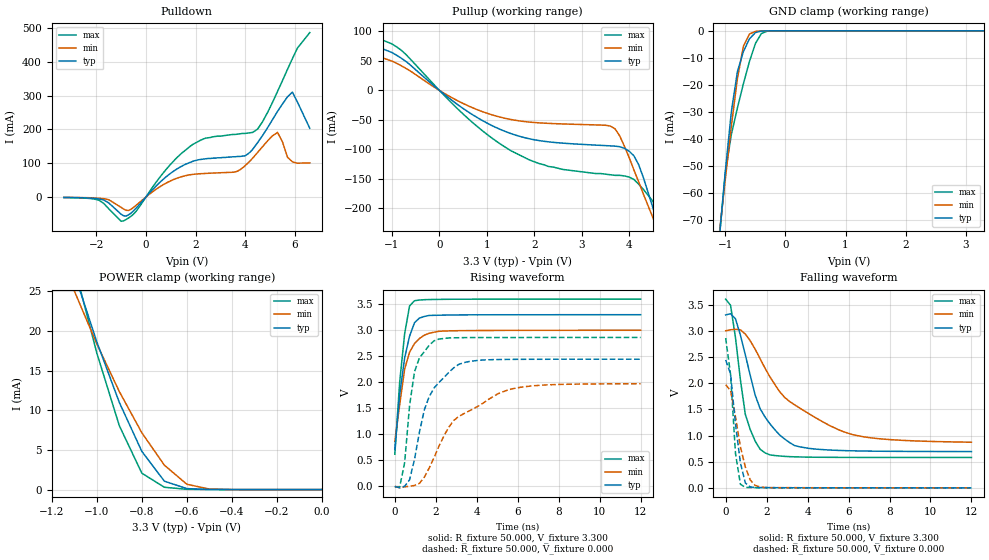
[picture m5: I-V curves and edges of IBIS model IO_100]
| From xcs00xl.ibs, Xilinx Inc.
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|   Model IO_100
[Model]   IO_100
Model_type   I/O
Polarity   Non-Inverting
Enable   Active-Low
Vinl =   0.800V
Vinh =   2.000V
Vmeas =   1.650V
Cref =  50.000pF
Rref =   1.000M
Vref =  0.000V
C_comp   5.300pF   3.500pF   6.800pF
[Temperature Range]   50.000   100.000   0.000
[Voltage Range]   3.300V   3.000V   3.600V
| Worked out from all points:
|   slope of the pulldown table from 0 to 0.495 V, typ, clamps not added: 12.8 ohm
|   slope of the pullup table from 0 to 0.495 V, typ, clamps not added: 16.3 ohm
|   GND clamp passes 1 mA (typ) near -0.52 V on its own axis
|   POWER clamp passes 1 mA (typ) near -0.69 V on its own axis
|   rising waveform, R_fixture 50.000, V_fixture 3.300: 20-80 % time 543ps typ, 571ps min, 408ps max; typ from 0.7 V to 3.3 V
|   rising waveform, R_fixture 50.000, V_fixture 0.000: 20-80 % time 1.12ns typ, 2.49ns min, 534ps max; typ from -0.012 V to 2.44 V
|   falling waveform, R_fixture 50.000, V_fixture 3.300: 20-80 % time 1.37ns typ, 3.04ns min, 712ps max; typ from 3.31 V to 0.694 V
|   falling waveform, R_fixture 50.000, V_fixture 0.000: 20-80 % time 421ps typ, 588ps min, 318ps max; typ from 2.44 V to 0.001 V
[Pulldown]
| voltage   I(typ)   I(min)   I(max)
-3.3V     -1.3mA     -1mA       -1.5mA
-1.9V     -5.4mA     -3.4mA     -9mA
-1V       -50.64mA   -30.43mA   -71.65mA
-700mV    -52.55mA   -39.74mA   -61.89mA
800mV     58.88mA    40.69mA    80.44mA
1.8V      103mA      66.09mA    151mA
3.6V      119mA      74.19mA    185mA
4V        122mA      93.03mA    188mA
4.5V      161mA      132mA      201mA
5.3V      253mA      191mA      312mA
5.9V      310mA      104mA      409mA
6.6V      203mA      101mA      486mA
[Pullup]
| voltage   I(typ)   I(min)   I(max)
-3.3V     5.1mA      940uA      37.2mA
-3.1V     7.54mA     1.17mA     90.7mA
-2.9V     27.6mA     1.66mA     104mA
-2.7V     86.4mA     3.45mA     105mA
-2.3V     90.2mA     70mA       105mA
-1.5V     80.17mA    63.43mA    95.35mA
-800mV    54.4mA     41.67mA    67.93mA
1.5V      -72.97mA   -49.19mA   -102mA
3.7V      -94.47mA   -64.95mA   -144mA
4.1V      -111mA     -135mA     -151mA
4.7V      -250mA     -255mA     -227mA
6.6V      -645mA     -572mA     -737mA
[GND_clamp]
| voltage   I(typ)   I(min)   I(max)
-3.3V     -539mA     -461mA     -635mA
-1.1V     -76.29mA   -74.81mA   -76.3mA
-1V       -51.66mA   -54.6mA    -52.25mA
-900mV    -29.77mA   -35.09mA   -38.23mA
-800mV    -15.1mA    -17.65mA   -28.49mA
-700mV    -7.645mA   -5.66mA    -19.53mA
-600mV    -2.968mA   -1.205mA   -11.34mA
-500mV    -649uA     -202uA     -4.68mA
-400mV    -83.34uA   -28.89uA   -976uA
-300mV    -8.303uA   -3.567uA   -95.2uA
3.3V      90.25nA    487nA      4.544uA
[POWER_clamp]
| voltage   I(typ)   I(min)   I(max)
-3.3V     51.86mA    10.89mA    181mA
-3.1V     70.08mA    13.61mA    230mA
-3V       85.17mA    15.89mA    249mA
-2.9V     108mA      19.33mA    255mA
-2.8V     138mA      24.96mA    249mA
-1.1V     27.32mA    25.08mA    28.22mA
-1V       18.65mA    18.39mA    17.25mA
-900mV    11mA       12.37mA    8.069mA
-800mV    4.821mA    7.171mA    2.071mA
-700mV    1.064mA    3.083mA    296uA
-600mV    127uA      671uA      39.67uA
0V        90.21nA    23.3nA     5.636uA
[Ramp]
| variable   typ   min   max
dV/dt_r   1.465/1.101n   1.181/2.487n   1.717/0.501n
dV/dt_f   1.563/1.371n   1.276/3.036n   1.811/0.692n
R_load = 50.000
[Rising Waveform]
R_fixture = 50.000
V_fixture = 3.300
V_fixture_min = 3.000
V_fixture_max = 3.600
L_fixture = 0.000H
C_fixture = 0.000F
| time   V(typ)   V(min)   V(max)
0s        700mV      857mV      612mV
240ps     1.771V     1.571V     2.013V
480ps     2.468V     2.252V     2.934V
720ps     2.885V     2.577V     3.468V
960ps     3.144V     2.743V     3.568V
1.2ns     3.234V     2.84V      3.582V
1.44ns    3.265V     2.904V     3.588V
1.68ns    3.285V     2.942V     3.591V
2.16ns    3.289V     2.979V     3.594V
12ns      3.299V     2.999V     3.599V
[Rising Waveform]
R_fixture = 50.000
V_fixture = 0.000
V_fixture_min = 0.000
V_fixture_max = 0.000
L_fixture = 0.000H
C_fixture = 0.000F
| time   V(typ)   V(min)   V(max)
0s        -11.88mV   -7.26mV    -16.02mV
240ps     -35.24mV   -37.87mV   -15.1mV
480ps     -7.661mV   -18.35mV   449mV
720ps     118mV      -5.72mV    1.547V
960ps     508mV      7.221mV    2.198V
1.44ns    1.465V     168mV      2.585V
1.92ns    1.889V     550mV      2.796V
2.88ns    2.276V     1.262V     2.854V
5.52ns    2.438V     1.849V     2.859V
12ns      2.441V     1.968V     2.861V
[Falling Waveform]
R_fixture = 50.000
V_fixture = 3.300
V_fixture_min = 3.000
V_fixture_max = 3.600
L_fixture = 0.000H
C_fixture = 0.000F
| time   V(typ)   V(min)   V(max)
0s        3.305V     3.003V     3.608V
240ps     3.33V      3.022V     3.49V
480ps     3.232V     3.031V     2.871V
960ps     2.544V     2.941V     1.406V
1.44ns    1.776V     2.651V     895mV
1.92ns    1.356V     2.289V     670mV
2.64ns    1.01V      1.837V     610mV
3.36ns    810mV      1.589V     594mV
5.76ns    713mV      1.073V     583mV
12ns      694mV      873mV      581mV
[Falling Waveform]
R_fixture = 50.000
V_fixture = 0.000
V_fixture_min = 0.000
V_fixture_max = 0.000
L_fixture = 0.000H
C_fixture = 0.000F
| time   V(typ)   V(min)   V(max)
0s        2.445V     1.971V     2.864V
240ps     2.18V      1.86V      2.166V
480ps     1.22V      1.359V     659mV
720ps     481mV      787mV      70.33mV
960ps     94.77mV    398mV      8.852mV
1.2ns     18.16mV    152mV      7.106mV
1.44ns    7.853mV    47.06mV    4.281mV
1.68ns    5.485mV    17.85mV    3.408mV
1.92ns    6.263mV    7.829mV    2.964mV
12ns      501uV      671uV      338uV
